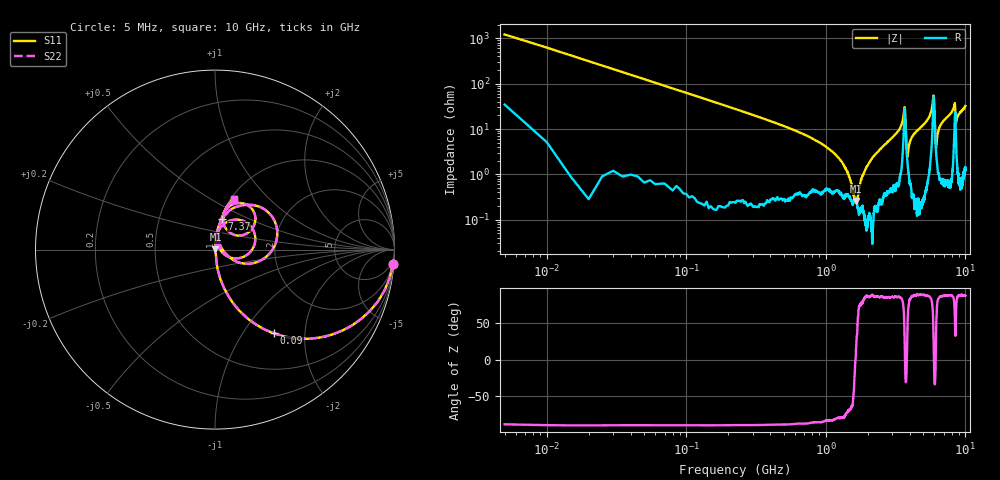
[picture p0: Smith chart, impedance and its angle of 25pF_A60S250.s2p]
! Amotech Co.,Ltd.
! http://www.amotech.co.kr/
! Part Number: A60S250
! These Parameters are Measured in Series Mode Connection
! Operation Temp=25[degC], DC Bias Voltage=0[V]
! Freq. Start=5[MHz] Stop=10[GHz], 2000[Steps]
! Date: Monday, July 13, 2020, 01:39:42
# GHZ S RI R 50.000000
!Freq.(Hz) S11(Real) S11(Imag) S21(Real) S21(Imag) S12(Real) S12(Imag) S22(Real) S22(Imag)
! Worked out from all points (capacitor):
!   2000 points, 5 MHz to 10 GHz, reference 50 ohm
!   read as one part in series: C = 25.3 pF near 55 MHz
!   lowest |Z| = 261 mohm at 1.655 GHz (marker M1)
!   series resonance near 1.633 GHz, so ESL is about 380 pH
!   S11 on the Smith chart (normalised r, x): 5 MHz: 2, -24; 90 MHz: 1.01, -1.40; 7.37 GHz: 1.01, +0.36; 10 GHz: 1.03, +0.64
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0.005  0.991 -0.0813  0.00901 0.0813  0.00901 0.0813  0.991 -0.0813
0.09  0.3285 -0.4663  0.6715 0.4663  0.6715 0.4663  0.3285 -0.4663
0.295  0.0436 -0.1991  0.9564 0.1991  0.9564 0.1991  0.0436 -0.1991
1.295  0.00388 -0.0187  0.9961 0.0187  0.9961 0.0187  0.00388 -0.0187
1.655  0.0024 0.00101  0.9976 -0.00101  0.9976 -0.00101  0.0024 0.00101
1.675  0.00242 0.00174  0.9976 -0.00174  0.9976 -0.00174  0.00242 0.00174
1.84  0.00184 0.00923  0.9982 -0.00923  0.9982 -0.00923  0.00184 0.00923
2.155  0.00083 0.0232  0.9992 -0.0232  0.9992 -0.0232  0.00083 0.0232
3.34  0.015 0.0924  0.985 -0.0924  0.985 -0.0924  0.015 0.0924
3.66  0.2072 0.1191  0.7928 -0.1191  0.7928 -0.1191  0.2072 0.1191
3.845  0.018 0.0163  0.982 -0.0163  0.982 -0.0163  0.018 0.0163
4.14  0.00749 0.0658  0.9925 -0.0658  0.9925 -0.0658  0.00749 0.0658
5.005  0.0176 0.1222  0.9824 -0.1222  0.9824 -0.1222  0.0176 0.1222
5.67  0.0728 0.2099  0.9272 -0.2099  0.9272 -0.2099  0.0728 0.2099
5.9  0.3304 0.1623  0.6696 -0.1623  0.6696 -0.1623  0.3304 0.1623
6  0.1831 -0.0789  0.8169 0.0789  0.8169 0.0789  0.1831 -0.0789
6.165  0.0301 0.0205  0.9699 -0.0205  0.9699 -0.0205  0.0301 0.0205
6.67  0.0229 0.1218  0.9771 -0.1218  0.9771 -0.1218  0.0229 0.1218
7.37  0.0373 0.1725  0.9627 -0.1725  0.9627 -0.1725  0.0373 0.1725
8.335  0.1567 0.2577  0.8433 -0.2577  0.8433 -0.2577  0.1567 0.2577
8.565  0.0701 0.1066  0.9299 -0.1066  0.9299 -0.1066  0.0701 0.1066
10  0.1036 0.2839  0.8964 -0.2839  0.8964 -0.2839  0.1036 0.2839
